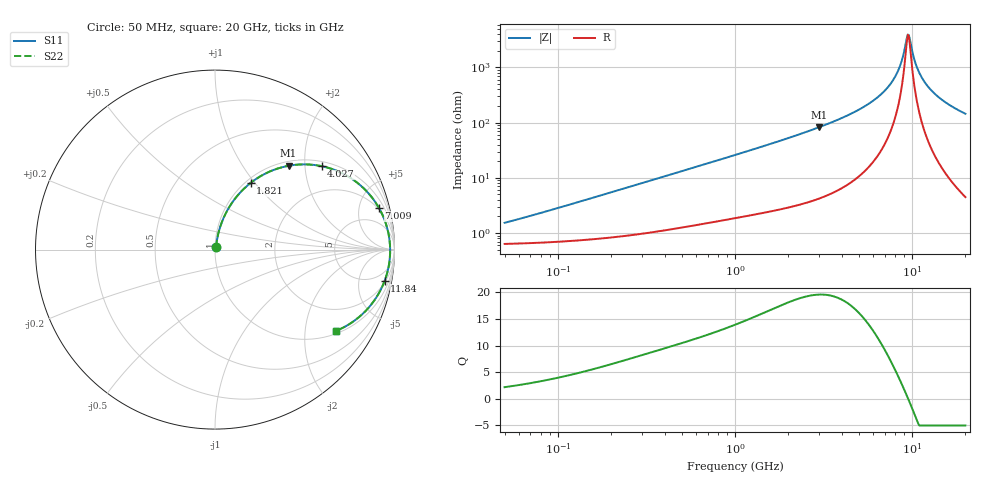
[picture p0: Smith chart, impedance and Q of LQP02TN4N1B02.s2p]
!Murata Part Number: LQP02TN4N1B02
!These Parameters are Measured in Series Mode Connection
!  o--[Z]--o
!Port1  Port2
!  o-------o
!Freq. Start=50[MHz] Stop=20[GHz], 401[Steps]
# Hz S RI R 50
!Freq.(Hz) S11(Real) S11(Imag) S21(Real) S21(Imag) S12(Real) S12(Imag) S22(Real) S22(Imag)
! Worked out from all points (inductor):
!   401 points, 50 MHz to 20 GHz, reference 50 ohm
!   read as one part in series: L = 4.4 nH near 71.63 MHz
!   highest Q = 19.6 at 2.985 GHz (marker M1), where L = 4.4 nH
!   self-resonance near 9.457 GHz
!   S11 on the Smith chart (normalised r, x): 50 MHz: 1.01, +0.03; 1.821 GHz: 1.05, +0.95; 4.027 GHz: 1.13, +2.44; 7.009 GHz: 1.82, +7.54; 11.84 GHz: 2, -11; 20 GHz: 1.09, -2.89
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5e7  0.0065 0.0138  0.9935 -0.0138  0.9935 -0.0138  0.0065 0.0138
1.364002e8  0.00873 0.0367  0.9913 -0.0367  0.9913 -0.0367  0.00873 0.0367
3.721004e8  0.02 0.0958  0.98 -0.0958  0.98 -0.0958  0.02 0.0958
1e9  0.0777 0.2341  0.9223 -0.2341  0.9223 -0.2341  0.0777 0.2341
1.820564e9  0.1979 0.371  0.8021 -0.371  0.8021 -0.371  0.1979 0.371
2.728004e9  0.3623 0.4557  0.6377 -0.4557  0.6377 -0.4557  0.3623 0.4557
2.98453e9  0.4102 0.467  0.5898 -0.467  0.5898 -0.467  0.4102 0.467
4.026975e9  0.5935 0.4651  0.4065 -0.4651  0.4065 -0.4651  0.5935 0.4651
5.515528e9  0.7938 0.3717  0.2062 -0.3717  0.2062 -0.3717  0.7938 0.3717
7.009217e9  0.913 0.2327  0.087 -0.2327  0.087 -0.2327  0.913 0.2327
7.442007e9  0.9344 0.1905  0.0656 -0.1905  0.0656 -0.1905  0.9344 0.1905
8.389408e9  0.9643 0.0998  0.0357 -0.0998  0.0357 -0.0998  0.9643 0.0998
8.774992e9  0.9708 0.0643  0.0292 -0.0643  0.0292 -0.0643  0.9708 0.0643
9.316812e9  0.9754 0.0163  0.0246 -0.0163  0.0246 -0.0163  0.9754 0.0163
9.457416e9  0.9757 0.00418  0.0243 -0.00418  0.0243 -0.00418  0.9757 0.00418
9.745021e9  0.9756 -0.02  0.0244 0.02  0.0244 0.02  0.9756 -0.02
1.019291e10  0.9731 -0.0562  0.0269 0.0562  0.0269 0.0562  0.9731 -0.0562
1.066139e10  0.9679 -0.0921  0.0321 0.0921  0.0321 0.0921  0.9679 -0.0921
1.183995e10  0.9455 -0.1733  0.0545 0.1733  0.0545 0.1733  0.9455 -0.1733
1.295331e10  0.9156 -0.2385  0.0844 0.2385  0.0844 0.2385  0.9156 -0.2385
1.460232e10  0.8621 -0.3164  0.1379 0.3164  0.1379 0.3164  0.8621 -0.3164
2e10  0.672 -0.4543  0.328 0.4543  0.328 0.4543  0.672 -0.4543
